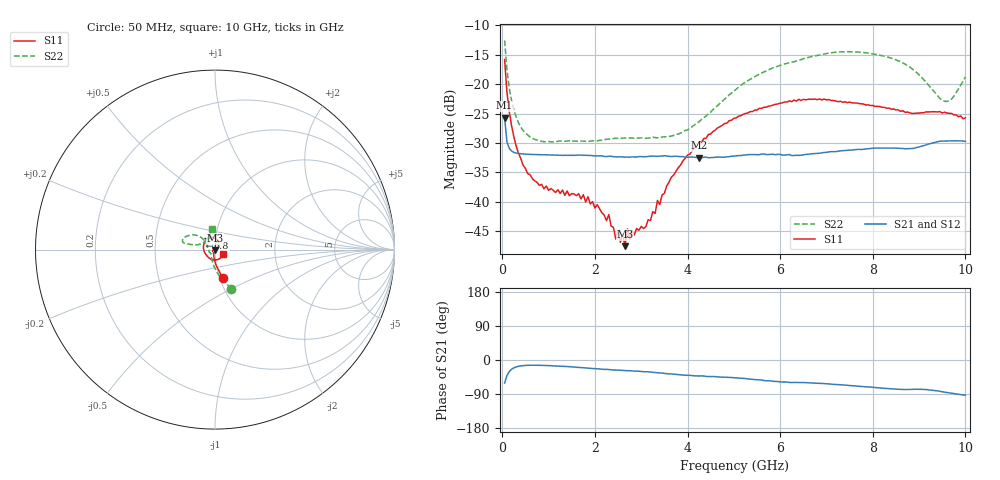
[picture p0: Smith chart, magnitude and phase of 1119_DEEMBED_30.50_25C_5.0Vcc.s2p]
!Hittite Microwave Corp.
!Digital Attenuator/PhaseShifter Rev 1.4.0
!Filename: C:\DATA\DATA\1119_DEEMBED_30.50_25C_5.0Vcc.s2p
!VNA ID: Agilent Technologies,N5224A,MY51441122,A.10.45.03
!Device type:
!2 Port Calibration.
!Temp(C): 25
!Lot Number:
!Serial Number:
!Operator:
!Misc:
!Attenuator:  30.500
# GHZ S DB R 50.0
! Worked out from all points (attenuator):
!   200 points, 50 MHz to 10 GHz, reference 50 ohm
!   highest |S21| = -25.69 dB at 50 MHz (marker M1); lowest = -32.5 dB at 4.25 GHz (marker M2)
!   lowest |S11| = -47.5 dB at 2.65 GHz (marker M3), VSWR 1.01, Z = 50 - j0.42 ohm
!   |S11| at or under -10 dB: start of sweep to end of sweep
!   |S22| runs from -29.8 to -12.6 dB; largest |S21 - S12| = 0.00012
!   S11 on the Smith chart (normalised r, x): 50 MHz: 1.03, -0.33; 6.8 GHz: 0.92, +0.12; 10 GHz: 1.10, -0.05
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0.05  -15.81 -75.0  -25.69 -60.7  -25.69 -60.7  -12.56 -67.5
0.1  -21.30 -86.3  -29.77 -41.3  -29.77 -41.4  -17.51 -84.0
0.2  -27.05 -97.5  -31.35 -24.3  -31.35 -24.5  -22.78 -100.6
0.55  -35.21 -122.1  -31.91 -14.1  -31.91 -14.0  -28.65 -126.5
0.9  -37.78 -136.1  -31.99 -14.4  -31.99 -14.4  -29.76 -135.9
1.75  -38.78 -143.1  -32.08 -20.5  -32.09 -20.5  -29.67 -140.9
2.25  -43.19 -131.4  -32.30 -24.6  -32.31 -24.6  -29.37 -148.0
2.3  -42.16 -136.3  -32.24 -25.1  -32.23 -25.2  -29.31 -149.4
2.45  -46.33 -122.3  -32.33 -26.4  -32.34 -26.5  -29.19 -151.0
2.5  -44.84 -112.8  -32.36 -26.8  -32.36 -26.9  -29.21 -151.6
2.65  -47.53 -92.1  -32.40 -27.8  -32.40 -27.8  -29.14 -154.2
2.7  -44.58 -76.0  -32.38 -28.3  -32.39 -28.3  -29.19 -154.5
2.75  -46.42 -74.5  -32.41 -28.3  -32.42 -28.4  -29.15 -155.6
3.4  -40.47 19.8  -32.22 -33.9  -32.23 -34.0  -29.06 -173.8
3.65  -35.80 35.4  -32.30 -36.8  -32.29 -36.9  -28.82 177.0
4.25  -30.00 50.3  -32.51 -42.3  -32.52 -42.2  -26.38 152.0
5.05  -25.73 71.8  -32.18 -47.0  -32.20 -47.1  -20.83 138.6
6.7  -22.58 118.9  -31.81 -60.7  -31.82 -60.7  -15.26 153.8
6.8  -22.63 121.9  -31.76 -61.5  -31.78 -61.5  -15.12 155.1
8.35  -24.06 -177.0  -30.87 -75.5  -30.87 -75.6  -15.45 168.1
9.55  -24.75 -77.3  -29.65 -84.9  -29.65 -84.9  -22.91 138.1
10  -25.72 -25.6  -29.72 -93.0  -29.71 -93.0  -18.76 98.2
